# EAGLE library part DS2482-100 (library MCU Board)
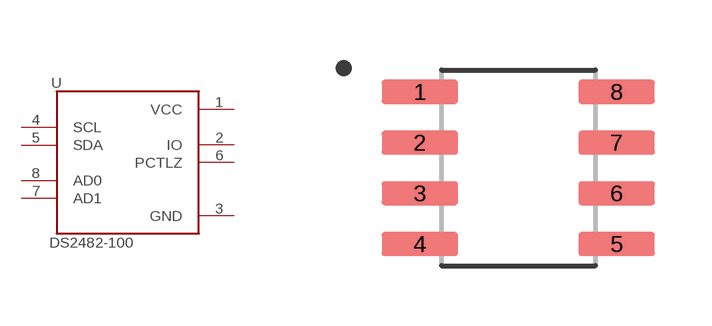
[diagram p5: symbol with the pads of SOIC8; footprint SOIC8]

Designator prefix U

## DS2482-100  [SOIC8]
1  VCC
2  IO
3  GND
4  SCL
5  SDA
6  PCTLZ
7  AD1
8  AD0

## Footprint SOIC8 (pad centres in mm)
smd 1.91 x 0.6: 1 -2.46,1.905; 2 -2.46,0.635; 3 -2.46,-0.635; 4 -2.46,-1.905; 5 2.46,-1.905; 6 2.46,-0.635; 7 2.46,0.635; 8 2.46,1.905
